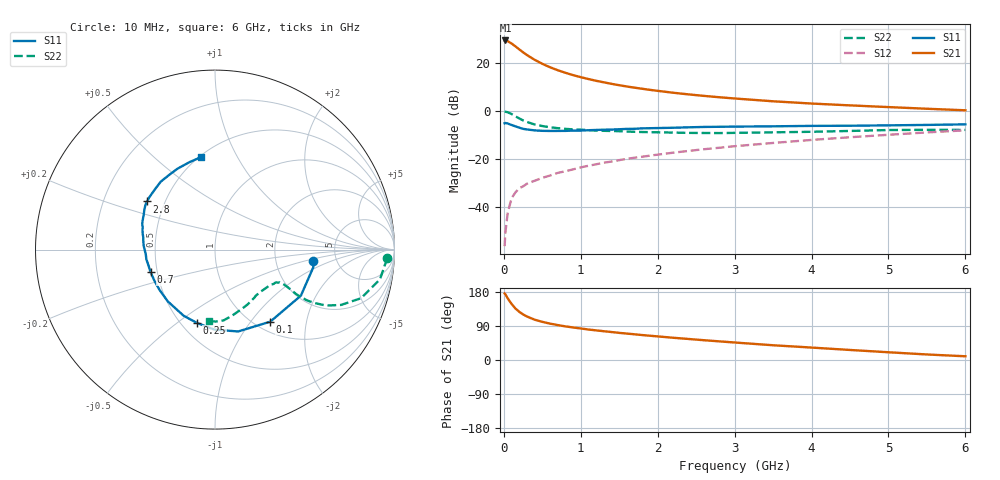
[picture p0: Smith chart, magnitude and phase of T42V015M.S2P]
! Infineon Technologies  Discrete & RF Semiconductors
! BFR182T
! Si NPN RF Bipolar Junction Transistor in SC75
! VCE = 2 V  IC = 15 mA
! Common Emitter S-Parameters:  October  1999
# GHz  S  MA  R  50
!  f  S11  S21  S12  S22
! GHz  MAG  ANG  MAG  ANG  MAG  ANG  MAG  ANG
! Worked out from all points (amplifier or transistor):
!   36 points, 10 MHz to 6 GHz, reference 50 ohm
!   highest |S21| = 29.3 dB at 20 MHz (marker M1)
!   |S21| within 3 dB of that: start of sweep to 171.7 MHz
!   unconditionally stable (mu >= 1): 711.1 MHz to 3.765 GHz
!   at 250 MHz: K = 0.61, MSG = 28.0 dB, |S12| = -31.5 dB
!   at 1.4 GHz: K = 1.13, MAG = 14.0 dB, |S12| = -21.2 dB
!   at 6 GHz: K = 0.85, MSG = 4.2 dB, |S12| = -8.1 dB
!   S11 on the Smith chart (normalised r, x): 10 MHz: 3.31, -0.62; 100 MHz: 1.16, -1.25; 250 MHz: 0.60, -0.59; 700 MHz: 0.46, -0.14; 2.8 GHz: 0.40, +0.27; 6 GHz: 0.51, +0.72
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0.01  0.549 -6.8  29.26 175.6  0.0015 83.7  0.9573 -2.8
0.02  0.5567 -10.1  29.32 173.2  0.0029 91.2  0.9549 -4.1
0.05  0.543 -28.2  28.3 162.7  0.0073 78.3  0.9339 -10.2
0.1  0.506 -52.5  25.34 148.1  0.015 73.6  0.8579 -18.4
0.15  0.4741 -74.2  22.09 136.1  0.0198 65.3  0.767 -23.7
0.2  0.4457 -90.5  19.14 127.2  0.0242 63.5  0.6939 -26.7
0.25  0.4205 -103.9  16.6 120.3  0.0265 59.6  0.6304 -28.2
0.3  0.408 -115.3  14.57 114.8  0.0301 60.5  0.5852 -28.9
0.4  0.3905 -132.3  11.59 106.4  0.0347 59.9  0.5185 -28.8
0.5  0.382 -144.2  9.563 100.7  0.0399 62.4  0.4807 -27.9
0.6  0.3795 -153.2  8.092 96.0  0.0446 63.3  0.4538 -27.3
0.7  0.3802 -160.6  7.032 92.2  0.0506 64.7  0.4342 -26.9
0.9  0.3861 -172.0  5.547 85.9  0.0599 67.0  0.4089 -26.9
1.1  0.3932 179.5  4.592 80.4  0.0714 68.2  0.3952 -27.7
1.3  0.4031 172.6  3.922 75.9  0.0828 69.2  0.382 -29.1
1.6  0.4193 164.6  3.211 69.7  0.0994 69.3  0.3688 -31.7
2.2  0.4429 153.7  2.383 58.7  0.1337 69.3  0.3512 -39.4
2.8  0.4639 144.7  1.918 49.2  0.1693 67.7  0.3428 -48.3
3.5  0.4744 134.8  1.578 38.9  0.2133 65.1  0.3554 -59.2
4.5  0.4878 122.1  1.297 26.5  0.2807 59.9  0.3798 -75.3
5.5  0.5075 106.3  1.103 14.6  0.3539 53.7  0.401 -89.3
6  0.5214 98.5  1.024 9.8  0.3916 49.6  0.3992 -95.1
